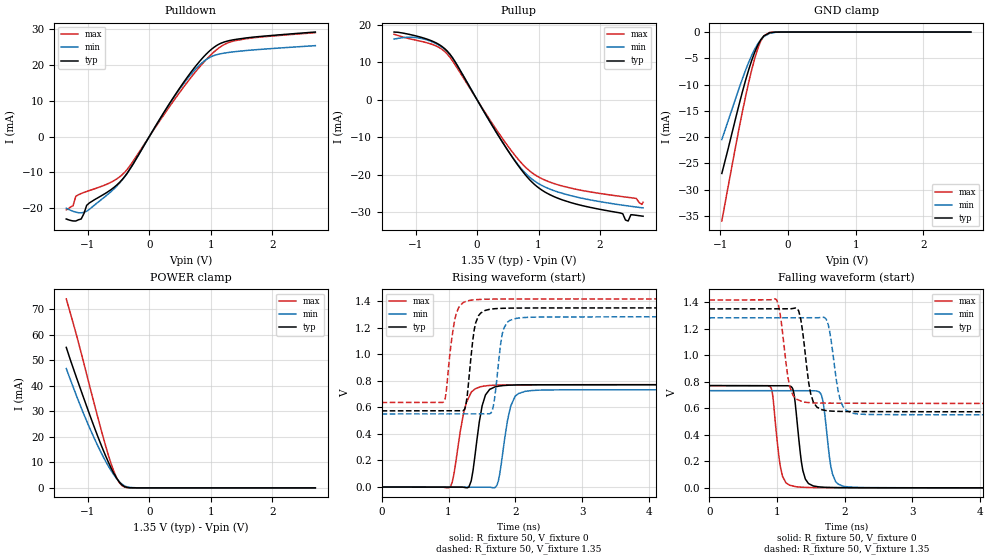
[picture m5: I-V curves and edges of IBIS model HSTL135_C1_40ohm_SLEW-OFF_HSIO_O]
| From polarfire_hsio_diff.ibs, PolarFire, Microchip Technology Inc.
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|   Model HSTL135_C1_40ohm_SLEW-OFF_HSIO_O
[Model]   HSTL135_C1_40ohm_SLEW-OFF_HSIO_O
Model_type   Output
Polarity   Non-Inverting
Enable   Active-High
Vmeas =   0.675
Cref =   5p
Rref =   50
Vref =   0.675
|   typ   min   max
C_comp_pullup   1.335e-12   1.335e-12   1.380e-12
C_comp_pulldown  1.335e-12   1.335e-12   1.380e-12
[Temperature Range]  25C   100C   -40C
[Voltage Range]  1.35   1.2825   1.4175
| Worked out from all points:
|   slope of the pulldown table from 0 to 0.203 V, typ, clamps not added: 35.1 ohm
|   slope of the pullup table from 0 to 0.203 V, typ, clamps not added: 35.8 ohm
|   GND clamp passes 1 mA (typ) near -0.37 V on its own axis
|   POWER clamp passes 1 mA (typ) near -0.43 V on its own axis
|   rising waveform, R_fixture 50, V_fixture 0: 20-80 % time 131ps typ, 139ps min, 158ps max; typ from 0 V to 0.771 V
|   rising waveform, R_fixture 50, V_fixture 1.35: 20-80 % time 101ps typ, 101ps min, 114ps max; typ from 0.574 V to 1.35 V
|   falling waveform, R_fixture 50, V_fixture 0: 20-80 % time 101ps typ, 104ps min, 98.3ps max; typ from 0.771 V to 0 V
|   falling waveform, R_fixture 50, V_fixture 1.35: 20-80 % time 116ps typ, 126ps min, 117ps max; typ from 1.35 V to 0.574 V
[GND Clamp]
| Voltage   I(typ)   I(min)   I(max)
-974.5mV  -26.9mA    -20.45mA   -35.95mA
-753mV    -15.48mA   -11.94mA   -20.52mA
-664.5mV  -11.06mA   -8.652mA   -14.74mA
-575.9mV  -7.072mA   -5.674mA   -9.445mA
-531.6mV  -5.316mA   -4.365mA   -7.064mA
-487.3mV  -3.767mA   -3.209mA   -4.927mA
-443mV    -2.466mA   -2.228mA   -3.102mA
-398.7mV  -1.449mA   -1.441mA   -1.67mA
-354.4mV  -738.4uA   -854uA     -712.2uA
-265.8mV  -117.5uA   -220.3uA   -58.64uA
-44.3mV   -274.4nA   -1.655uA   -83.21nA
2.7V      0A         0A         0A
[POWER Clamp]
| Voltage   I(typ)   I(min)   I(max)
-1.35V    55.07mA    46.77mA    74.1mA
-1.196V   44.05mA    36.84mA    60.94mA
-974.5mV  29.03mA    23.74mA    40.36mA
-797.3mV  17.68mA    14.49mA    24.04mA
-664.5mV  10.01mA    8.483mA    12.73mA
-575.9mV  5.63mA     5.093mA    6.421mA
-531.6mV  3.786mA    3.641mA    3.935mA
-487.3mV  2.262mA    2.398mA    2.056mA
-443mV    1.133mA    1.41mA     851.4uA
-354.4mV  127.5uA    344.8uA    50.77uA
-221.5mV  1.715uA    33.09uA    747.7nA
2.7V      0A         0A         0A
[Pullup]
| Voltage   I(typ)   I(min)   I(max)
-1.35V    18.04mA    16.16mA    17.46mA
-885.9mV  16.53mA    16.25mA    15.48mA
-487.3mV  13.01mA    12.85mA    12.23mA
-354.4mV  10.03mA    10.04mA    9.253mA
548.4mV   -14.7mA    -14.66mA   -13.38mA
801.6mV   -20.34mA   -19.83mA   -18.19mA
1.012V    -23.61mA   -22.47mA   -20.69mA
1.527V    -27.42mA   -25.57mA   -23.55mA
2.369V    -30.37mA   -28.09mA   -25.83mA
2.457V    -32.31mA   -28.3mA    -26.01mA
2.502V    -30.63mA   -28.39mA   -26.11mA
2.7V      -31.04mA   -28.82mA   -27.32mA
[Pulldown]
| Voltage   I(typ)   I(min)   I(max)
-1.35V    -23.02mA   -20.03mA   -20.47mA
-1.24V    -23.57mA   -20.86mA   -19.32mA
-1.196V   -23.58mA   -21.11mA   -16.72mA
-1.063V   -21.53mA   -21.18mA   -15.61mA
-974.5mV  -18.54mA   -20.32mA   -15.08mA
-531.6mV  -13.58mA   -13.88mA   -11.85mA
-354.4mV  -10.11mA   -10.12mA   -9.082mA
548.4mV   14.91mA    14.58mA    13.61mA
843.8mV   21.52mA    20.41mA    19.96mA
1.055V    24.98mA    22.65mA    23.69mA
1.394V    27.13mA    23.73mA    26.8mA
2.7V      29.21mA    25.41mA    29.03mA
[Ramp]
dV/dt_r   0.462738/0.131441n  0.439991/0.138968n  0.462765/0.158087n
dV/dt_f   0.465721/0.116446n  0.438941/0.126488n  0.468357/0.11705n
R_load = 50
[Rising Waveform]
R_fixture = 50
V_fixture = 0
V_fixture_min = 0
V_fixture_max = 0
| Time   V(typ)   V(min)   V(max)
0s        1.383uV    1.564uV    2.106uV
1.029ns   -463.2uV   -601.7uV   2.793mV
1.22ns    -1.422mV   -713.7uV   544mV
1.304ns   -246.9uV   -763uV     676.2mV
1.366ns   123.4mV    -799.3uV   726.4mV
1.525ns   649.1mV    -892.5uV   760.3mV
1.722ns   757.1mV    11.93mV    768.1mV
1.929ns   767.7mV    609.7mV    769.9mV
2.149ns   769.7mV    721.5mV    770.2mV
10ns      771.2mV    733.3mV    771.3mV
[Rising Waveform]
R_fixture = 50
V_fixture = 1.35
V_fixture_min = 1.2825
V_fixture_max = 1.4175
| Time   V(typ)   V(min)   V(max)
0s        573.8mV    550.9mV    636.9mV
930ps     574.5mV    551.1mV    643.1mV
1.098ns   574.7mV    551.2mV    1.271V
1.243ns   589.1mV    551.2mV    1.395V
1.313ns   859.9mV    551.2mV    1.406V
1.45ns    1.292V     551.3mV    1.413V
1.649ns   1.341V     570.5mV    1.416V
1.802ns   1.346V     1.151V     1.416V
2ns       1.348V     1.269V     1.416V
10ns      1.35V      1.282V     1.417V
[Falling Waveform]
R_fixture = 50
V_fixture = 0
V_fixture_min = 0
V_fixture_max = 0
| Time   V(typ)   V(min)   V(max)
0s        771.2mV    733.3mV    771.3mV
902ps     770.5mV    732.9mV    761.8mV
1.082ns   770.4mV    732.9mV    87.53mV
1.228ns   751.9mV    732.8mV    14.95mV
1.282ns   577.7mV    732.8mV    8.265mV
1.42ns    65.59mV    732.7mV    3.776mV
1.655ns   5.947mV    701.1mV    1.567mV
1.819ns   2.475mV    107.8mV    1.165mV
1.981ns   1.569mV    11.99mV    941.5uV
10ns      2.06uV     3.194uV    7.381uV
[Falling Waveform]
R_fixture = 50
V_fixture = 1.35
V_fixture_min = 1.2825
V_fixture_max = 1.4175
| Time   V(typ)   V(min)   V(max)
0s        1.35V      1.282V     1.417V
996ps     1.351V     1.283V     1.417V
1.19ns    1.351V     1.283V     761.1mV
1.322ns   1.333V     1.283V     661.8mV
1.387ns   1.147V     1.283V     647.9mV
1.538ns   646.5mV    1.283V     641.2mV
1.744ns   581.7mV    1.254V     639.1mV
1.932ns   576.7mV    669.8mV    638.7mV
2.11ns    575.7mV    563.8mV    638.3mV
10ns      573.8mV    550.9mV    636.9mV
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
